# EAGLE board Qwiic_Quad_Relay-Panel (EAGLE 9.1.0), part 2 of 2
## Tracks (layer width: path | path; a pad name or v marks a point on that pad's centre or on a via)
3.3V  (via drill 0.35)
  Top 0.254: J3.2 13.6,43.04 v13.84,42.8
  Top 0.305: J2.2 83.32,42.04 v82.93,41.66
  Bottom 0.305: v13.84,42.8 13.84,39.24 16.26,36.83 17.78,36.83 18.41,37.46 33.78,37.46 34.42,36.83 36.07,36.83 37.34,38.1 53.59,38.1 55.37,36.32 56.77,36.32 58.29,37.85 74.68,37.85 75.69,36.83 79.5,36.83 82.93,40.26 v82.93,41.66
3.3V1  (via drill 0.35)
  Top 0.254: J11.2 96.66,43.04 v96.9,42.8
  Top 0.305: J10.2 166.38,42.04 v165.99,41.66
  Bottom 0.305: v96.9,42.8 96.9,39.24 99.31,36.83 100.84,36.83 101.47,37.46 116.84,37.46 117.48,36.83 119.13,36.83 120.4,38.1 136.65,38.1 138.43,36.32 139.83,36.32 141.35,37.85 157.73,37.85 158.75,36.83 162.56,36.83 165.99,40.26 v165.99,41.66
3.3V2  (via drill 0.35)
  Top 0.254: J20.2 13.6,90.54 v13.84,90.3
  Top 0.305: J19.2 83.32,89.54 v82.93,89.15
  Bottom 0.305: v13.84,90.3 13.84,86.74 16.26,84.33 17.78,84.33 18.41,84.96 33.78,84.96 34.42,84.33 36.07,84.33 37.34,85.6 53.59,85.6 55.37,83.82 56.77,83.82 58.29,85.34 74.68,85.34 75.69,84.33 79.5,84.33 82.93,87.76 v82.93,89.15
3.3V3  (via drill 0.35)
  Top 0.254: J29.2 96.66,90.54 v96.9,90.3
  Top 0.305: J28.2 166.38,89.54 v165.99,89.15
  Bottom 0.305: v96.9,90.3 96.9,86.74 99.31,84.33 100.84,84.33 101.47,84.96 116.84,84.96 117.48,84.33 119.13,84.33 120.4,85.6 136.65,85.6 138.43,83.82 139.83,83.82 141.35,85.34 157.73,85.34 158.75,84.33 162.56,84.33 165.99,87.76 v165.99,89.15
5V  (via drill 0.51)
  Top 0.254: 61.23,38.1 52.16,38.1 | 52.16,38.1 44.45,38.1 | R8.1 44.45,38.61 44.45,38.35 44.45,38.1 | 22.35,38.61 13.21,38.61 12.66,38.06 R1.2 | D9.A 83.31,37.72 82.42,38.61 72.77,38.61 72.52,38.35 72.48,38.31 72.48,37.97 | D2.A 22.35,38.61 | J4.2 35.05,43.56 34.16,42.67 U5.1 34.2,41.99 C1.1 34.2,38.65 34.16,38.61 | D3.A 64.39,50.93 64.14,50.67 64.14,47.5 64.01,47.37 | U1.2 59.56,41.95 | 59.56,41.95 R6.2 | 59.56,41.95 59.6,41.91 60.58,41.91 61.23,41.26 61.23,38.61 61.23,38.35 61.23,38.1 | R14.2 72.48,37.97 | R13.2 52.16,38.1 | 44.45,38.1 42.67,38.1 | 42.67,38.1 36.2,38.1 35.69,38.61 34.16,38.61 | 34.16,38.61 31.88,38.61 | 31.88,38.61 31.75,38.61 | 31.75,38.61 28.57,38.61 28.07,38.1 24.13,38.1 23.62,38.61 22.35,38.61 | R12.2 31.84,38.52 31.75,38.61 | 31.88,38.61 31.84,38.65 R5.2 | D7.A 42.67,38.1 | 61.23,38.1 62.99,38.1 | 62.99,38.1 63.25,38.1 64.01,37.34 70.48,37.34 70.99,37.85 72.35,37.85 72.48,37.97 | D8.A 62.99,38.1
  Top 0.508: C3.1 C2.1 66.08,47.37 64.01,47.37 60.83,47.37 v60.26,46.8 59.56,46.1 U1.2
  Bottom 0.254: J1.3 34.16,49.4 34.16,46.35 35.69,44.83 35.69,43.81 J4.2
  Bottom 0.508: JP7.2 63.75,43.31 v60.26,46.8
5V1  (via drill 0.51)
  Top 0.254: 144.28,38.1 135.22,38.1 | 135.22,38.1 127.51,38.1 | R21.1 127.51,38.61 127.51,38.35 127.51,38.1 | 105.41,38.61 96.27,38.61 95.72,38.06 R18.2 | D19.A 166.37,37.72 165.48,38.61 155.83,38.61 155.58,38.35 155.54,38.31 155.54,37.97 | D12.A 105.41,38.61 | J12.2 118.11,43.56 117.22,42.67 U7.1 117.26,41.99 C5.1 117.26,38.65 117.22,38.61 | D13.A 147.45,50.93 147.19,50.67 147.19,47.5 147.07,47.37 | U8.2 142.62,41.95 | 142.62,41.95 R33.2 | 142.62,41.95 142.66,41.91 143.64,41.91 144.28,41.26 144.28,38.61 144.28,38.35 144.28,38.1 | R29.2 155.54,37.97 | R28.2 135.22,38.1 | 127.51,38.1 125.73,38.1 | 125.73,38.1 119.25,38.1 118.75,38.61 117.22,38.61 | 117.22,38.61 114.94,38.61 | 114.94,38.61 114.81,38.61 | 114.81,38.61 111.63,38.61 111.12,38.1 107.19,38.1 106.68,38.61 105.41,38.61 | R27.2 114.9,38.52 114.81,38.61 | 114.94,38.61 114.9,38.65 R20.2 | D17.A 125.73,38.1 | 144.28,38.1 146.05,38.1 | 146.05,38.1 146.3,38.1 147.07,37.34 153.54,37.34 154.05,37.85 155.41,37.85 155.54,37.97 | D18.A 146.05,38.1
  Top 0.508: C7.1 C6.1 149.14,47.37 147.07,47.37 143.89,47.37 v143.32,46.8 142.62,46.1 U8.2
  Bottom 0.254: J14.3 117.22,49.4 117.22,46.35 118.75,44.83 118.75,43.81 J12.2
  Bottom 0.508: JP18.2 146.81,43.31 v143.32,46.8
5V2  (via drill 0.51)
  Top 0.254: 61.23,85.6 52.16,85.6 | 52.16,85.6 44.45,85.6 | R38.1 44.45,86.11 44.45,85.85 44.45,85.6 | 22.35,86.11 13.21,86.11 12.66,85.56 R35.2 | D29.A 83.31,85.22 82.42,86.11 72.77,86.11 72.52,85.85 72.48,85.81 72.48,85.47 | D22.A 22.35,86.11 | J21.2 35.05,91.06 34.16,90.17 U11.1 34.2,89.49 C9.1 34.2,86.15 34.16,86.11 | D23.A 64.39,98.42 64.14,98.17 64.14,95 64.01,94.87 | U12.2 59.56,89.45 | 59.56,89.45 R50.2 | 59.56,89.45 59.6,89.41 60.58,89.41 61.23,88.76 61.23,86.11 61.23,85.85 61.23,85.6 | R46.2 72.48,85.47 | R45.2 52.16,85.6 | 44.45,85.6 42.67,85.6 | 42.67,85.6 36.2,85.6 35.69,86.11 34.16,86.11 | 34.16,86.11 31.88,86.11 | 31.88,86.11 31.75,86.11 | 31.75,86.11 28.57,86.11 28.07,85.6 24.13,85.6 23.62,86.11 22.35,86.11 | R44.2 31.84,86.02 31.75,86.11 | 31.88,86.11 31.84,86.15 R37.2 | D27.A 42.67,85.6 | 61.23,85.6 62.99,85.6 | 62.99,85.6 63.25,85.6 64.01,84.84 70.48,84.84 70.99,85.34 72.35,85.34 72.48,85.47 | D28.A 62.99,85.6
  Top 0.508: C11.1 C10.1 66.08,94.87 64.01,94.87 60.83,94.87 v60.26,94.3 59.56,93.6 U12.2
  Bottom 0.254: J23.3 34.16,96.9 34.16,93.85 35.69,92.33 35.69,91.31 J21.2
  Bottom 0.508: JP27.2 63.75,90.81 v60.26,94.3
5V3  (via drill 0.51)
  Top 0.254: 144.28,85.6 135.22,85.6 | 135.22,85.6 127.51,85.6 | R55.1 127.51,86.11 127.51,85.85 127.51,85.6 | 105.41,86.11 96.27,86.11 95.72,85.56 R52.2 | D39.A 166.37,85.22 165.48,86.11 155.83,86.11 155.58,85.85 155.54,85.81 155.54,85.47 | D32.A 105.41,86.11 | J30.2 118.11,91.06 117.22,90.17 U15.1 117.26,89.49 C13.1 117.26,86.15 117.22,86.11 | D33.A 147.45,98.42 147.19,98.17 147.19,95 147.07,94.87 | U16.2 142.62,89.45 | 142.62,89.45 R67.2 | 142.62,89.45 142.66,89.41 143.64,89.41 144.28,88.76 144.28,86.11 144.28,85.85 144.28,85.6 | R63.2 155.54,85.47 | R62.2 135.22,85.6 | 127.51,85.6 125.73,85.6 | 125.73,85.6 119.25,85.6 118.75,86.11 117.22,86.11 | 117.22,86.11 114.94,86.11 | 114.94,86.11 114.81,86.11 | 114.81,86.11 111.63,86.11 111.12,85.6 107.19,85.6 106.68,86.11 105.41,86.11 | R61.2 114.9,86.02 114.81,86.11 | 114.94,86.11 114.9,86.15 R54.2 | D37.A 125.73,85.6 | 144.28,85.6 146.05,85.6 | 146.05,85.6 146.3,85.6 147.07,84.84 153.54,84.84 154.05,85.34 155.41,85.34 155.54,85.47 | D38.A 146.05,85.6
  Top 0.508: C15.1 C14.1 149.14,94.87 147.07,94.87 143.89,94.87 v143.32,94.3 142.62,93.6 U16.2
  Bottom 0.254: J32.3 117.22,96.9 117.22,93.85 118.75,92.33 118.75,91.31 J30.2
  Bottom 0.508: JP36.2 146.81,90.81 v143.32,94.3
!RESET
  Top 0.254: U5.4 37.97,42.41 37.08,43.3 37.08,44.2 38.35,45.47 39.88,45.47 J4.5 44.28,46.1 R8.2
!RESET1
  Top 0.254: U7.4 121.03,42.41 120.14,43.3 120.14,44.2 121.41,45.47 122.94,45.47 J12.5 127.34,46.1 R21.2
!RESET2
  Top 0.254: U11.4 37.97,89.91 37.08,90.8 37.08,91.69 38.35,92.96 39.88,92.96 J21.5 44.28,93.6 R38.2
!RESET3
  Top 0.254: U15.4 121.03,89.91 120.14,90.8 120.14,91.69 121.41,92.96 122.94,92.96 J30.5 127.34,93.6 R55.2
COM1
  Top 1.778: K1.4 13.21,20.83 15.24,18.8 15.75,18.8 20.45,18.8 23.5,15.75 J5.2
  Bottom 1.778: K1.4 13.21,20.83 15.24,18.8 20.49,18.8 J5.2
COM2
  Top 1.778: K2.4 33.53,20.32 35.31,18.54 37.13,18.54 J6.2
  Bottom 1.778: K2.4 33.53,20.32 35.31,18.54 37.13,18.54 J6.2 | J6.2
COM3
  Top 1.778: K3.4 53.85,18.29 56.31,15.83 J7.2
  Bottom 1.778: K3.4 53.85,18.29 56.31,15.83 J7.2
COM4
  Top 1.778: K4.4 74.17,17.23 J8.2 | K4.4
  Bottom 1.778: K4.4 74.17,17.23 J8.2 | K4.4
COM5
  Top 1.778: K5.4 96.27,20.83 98.3,18.8 98.81,18.8 103.51,18.8 106.55,15.75 J13.2
  Bottom 1.778: K5.4 96.27,20.83 98.3,18.8 103.55,18.8 J13.2
COM6
  Top 1.778: K6.4 116.59,20.32 118.36,18.54 120.19,18.54 J15.2
  Bottom 1.778: K6.4 116.59,20.32 118.36,18.54 120.19,18.54 J15.2 | J15.2
COM7
  Top 1.778: K7.4 136.91,18.29 139.37,15.83 J16.2
  Bottom 1.778: K7.4 136.91,18.29 139.37,15.83 J16.2
COM8
  Top 1.778: K8.4 157.23,17.23 J17.2 | K8.4
  Bottom 1.778: K8.4 157.23,17.23 J17.2 | K8.4
COM9
  Top 1.778: K9.4 13.21,68.33 15.24,66.29 15.75,66.29 20.45,66.29 23.5,63.25 J22.2
  Bottom 1.778: K9.4 13.21,68.33 15.24,66.29 20.49,66.29 J22.2
COM10
  Top 1.778: K10.4 33.53,67.82 35.31,66.04 37.13,66.04 J24.2
  Bottom 1.778: K10.4 33.53,67.82 35.31,66.04 37.13,66.04 J24.2 | J24.2
COM11
  Top 1.778: K11.4 53.85,65.79 56.31,63.33 J25.2
  Bottom 1.778: K11.4 53.85,65.79 56.31,63.33 J25.2
COM12
  Top 1.778: K12.4 74.17,64.72 J26.2 | K12.4
  Bottom 1.778: K12.4 74.17,64.72 J26.2 | K12.4
COM13
  Top 1.778: K13.4 96.27,68.33 98.3,66.29 98.81,66.29 103.51,66.29 106.55,63.25 J31.2
  Bottom 1.778: K13.4 96.27,68.33 98.3,66.29 103.55,66.29 J31.2
COM14
  Top 1.778: K14.4 116.59,67.82 118.36,66.04 120.19,66.04 J33.2
  Bottom 1.778: K14.4 116.59,67.82 118.36,66.04 120.19,66.04 J33.2 | J33.2
COM15
  Top 1.778: K15.4 136.91,65.79 139.37,63.33 J34.2
  Bottom 1.778: K15.4 136.91,65.79 139.37,63.33 J34.2
COM16
  Top 1.778: K16.4 157.23,64.72 J35.2 | K16.4
  Bottom 1.778: K16.4 157.23,64.72 J35.2 | K16.4
GND  (via drill 0.3)
  other vias: 53.34,36.96 73.53,36.83 32.77,36.45 13.97,37.34 71.37,36.83 86.11,37.08 50.8,36.96 11.43,37.34 30.86,36.45 38.48,40.64
  pour Bottom: 6.86,32.77 89.41,32.77 89.41,53.85 6.86,53.85
  pour Top: 6.86,32.77 6.86,53.85 89.41,53.85 89.41,32.77
GND1  (via drill 0.3)
  other vias: 136.4,36.96 156.59,36.83 115.82,36.45 97.03,37.34 154.43,36.83 169.16,37.08 133.86,36.96 94.49,37.34 113.92,36.45 121.54,40.64
  pour Bottom: 89.92,32.77 172.47,32.77 172.47,53.85 89.92,53.85
  pour Top: 89.92,32.77 89.92,53.85 172.47,53.85 172.47,32.77
GND2  (via drill 0.3)
  other vias: 53.34,84.45 73.53,84.33 32.77,83.95 13.97,84.84 71.37,84.33 86.11,84.58 50.8,84.45 11.43,84.84 30.86,83.95 38.48,88.14
  pour Bottom: 6.86,80.26 89.41,80.26 89.41,101.35 6.86,101.35
  pour Top: 6.86,80.26 6.86,101.35 89.41,101.35 89.41,80.26
GND3  (via drill 0.3)
  other vias: 136.4,84.45 156.59,84.33 115.82,83.95 97.03,84.84 154.43,84.33 169.16,84.58 133.86,84.45 94.49,84.84 113.92,83.95 121.54,88.14
  pour Bottom: 89.92,80.26 172.47,80.26 172.47,101.35 89.92,101.35
  pour Top: 89.92,80.26 89.92,101.35 172.47,101.35 172.47,80.26
MISO  (via drill 0.35)
  Top 0.254: U5.8 v41.78,49.02
  Bottom 0.254: v41.78,49.02 40,47.24 35.94,47.24 35.43,46.74 J4.1
MISO1  (via drill 0.35)
  Top 0.254: U7.8 v124.84,49.02
  Bottom 0.254: v124.84,49.02 123.06,47.24 119,47.24 118.49,46.74 J12.1
MISO2  (via drill 0.35)
  Top 0.254: U11.8 v41.78,96.52
  Bottom 0.254: v41.78,96.52 40,94.74 35.94,94.74 35.43,94.23 J21.1
MISO3  (via drill 0.35)
  Top 0.254: U15.8 v124.84,96.52
  Bottom 0.254: v124.84,96.52 123.06,94.74 119,94.74 118.49,94.23 J30.1
N$1
  Top 0.254: K2.5 41.4,22.1 38.61,24.89 38.61,31.88 37.85,32.64 37.72,32.77 30.1,32.77 29.84,33.03 D6.C 29.84,34.75 R12.1
N$2
  Top 0.254: D1.A 15.58,33.53 Q4.3 15.92,33.53 R4.1 25.06,30.57 K1.1
N$3
  Top 0.254: U3.3 25.27,44.45 25.65,44.07 27.94,44.07 28.96,43.05 31.5,43.05 31.88,43.43 R11.1
N$4
  Top 0.508: U1.3 61.87,41.25 62.99,40.13 63.63,39.5 D11.C 65.16,40.78 65.53,41.15 C4.A
N$5
  Top 0.254: R10.1 28.66,44.11 27.81,44.96 U3.1
N$6  (via drill 0.35)
  Top 0.254: U3.6 25.27,43.31 25.53,43.56 27.56,43.56 27.81,43.31 U3.8 27.81,41.27 28.57,40.51 v28.96,40.51 R5.1 | 51.94,43.18 53.85,43.18 54.1,43.18 54.48,42.8 U2.8 | U2.6 51.94,43.18 | v48.39,40.64 48.39,41.4 50.16,43.18 51.94,43.18
  Bottom 0.254: v48.39,40.64 47.75,40 29.46,40 v28.96,40.51
N$7
  Top 0.254: R1.1 10.79,34.88 D1.C 10.79,33.03 11.05,32.77 17.65,32.77 18.29,32.13 18.29,25.4 19.05,24.64 23.37,24.64 K1.5
N$8
  Top 0.254: R4.2 26.79,33.55 26.79,34.17 26.54,34.42 22.61,34.42 22.35,34.67 D2.C
N$9
  Top 0.254: U2.1 54.48,44.45 53.72,43.69 49.91,43.69 49.02,42.8 47.12,42.8 46.48,43.43 R2.1
N$10
  Top 0.254: D10.A 98.64,33.53 Q5.3 98.98,33.53 R19.1 108.12,30.57 K5.1
N$11
  Top 0.254: U2.3 51.94,45.08 51.09,44.23 R3.1
N$12
  Top 0.254: K2.1 45.38,30.57 R15.1 34.97,33.53 Q3.3 34.63,33.53 D6.A
N$13
  Top 0.254: D3.C 67.82,50.91 67.82,50.04 67.69,49.91 66.42,49.91 66.21,49.7 R9.1
N$14
  Top 0.254: R13.1 50.16,34.75 D4.C 50.16,33.03 50.42,32.77 58.04,32.77 58.93,31.88 | 58.93,31.88 58.93,23.5 60.26,22.16 60.32,22.1 K3.5 | 58.93,31.88 arc90 58.93,31.88
N$15
  Top 0.254: D4.A 54.95,33.53 Q2.3 55.29,33.53 R16.1 65.7,30.57 K3.1
N$16
  Top 0.254: 79.12,23.5 80.52,22.1 K4.5 | R14.1 70.48,34.88 D5.C 70.48,33.02 70.74,32.77 78.49,32.77 79.12,32.13 79.12,23.5 | 79.12,23.5
N$17
  Top 0.254: D5.A 75.27,33.53 Q1.3 75.61,33.53 R17.1 86.02,29.72 K4.1
N$18
  Top 0.254: R18.1 93.85,34.88 D10.C 93.85,33.03 94.11,32.77 100.71,32.77 101.35,32.13 101.35,25.4 102.11,24.64 106.43,24.64 K5.5
N$19
  Top 0.254: U1.1 57.25,43.24 57.82,42.67 R6.1 R7.2
N$20
  Top 0.254: R17.2 87.75,33.55 87.76,33.57 87.76,34.16 87.5,34.42 83.57,34.42 83.31,34.67 D9.C
N$21
  Top 0.254: R16.2 67.42,33.55 67.42,34.17 67.18,34.42 63.25,34.42 62.99,34.67 D8.C
N$22
  Top 0.254: D7.C 42.67,34.67 42.93,34.42 46.86,34.42 47.08,34.2 R15.2
N$23
  Top 0.254: R19.2 109.84,33.55 109.84,34.17 109.6,34.42 105.66,34.42 105.41,34.67 D12.C
N$24
  Top 0.254: D13.C 150.88,50.91 150.88,50.04 150.75,49.91 149.48,49.91 149.26,49.7 R22.1
N$25
  Top 0.254: U4.3 108.33,44.45 108.71,44.07 111,44.07 112.01,43.05 114.55,43.05 114.94,43.43 R26.1
N$26
  Top 0.254: R25.1 111.72,44.11 110.87,44.96 U4.1
N$27  (via drill 0.35)
  Top 0.254: U4.6 108.33,43.31 108.59,43.56 110.62,43.56 110.87,43.31 U4.8 110.87,41.27 111.63,40.51 v112.01,40.51 R20.1 | 135,43.18 136.91,43.18 137.16,43.18 137.54,42.8 U6.8 | U6.6 135,43.18 | v131.44,40.64 131.44,41.4 133.22,43.18 135,43.18
  Bottom 0.254: v131.44,40.64 130.81,40 112.52,40 v112.01,40.51
N$28
  Top 0.254: U6.1 137.54,44.45 136.78,43.69 132.97,43.69 132.08,42.8 130.17,42.8 129.54,43.43 R23.1
N$29
  Top 0.254: U6.3 135,45.08 134.15,44.23 R24.1
N$30
  Top 0.254: K6.5 124.46,22.1 121.67,24.89 121.67,31.88 120.9,32.64 120.78,32.77 113.16,32.77 112.9,33.03 D16.C 112.9,34.75 R27.1
N$31
  Top 0.254: K6.1 128.44,30.57 R30.1 118.03,33.53 Q8.3 117.69,33.53 D16.A
N$32
  Top 0.254: R28.1 133.22,34.75 D14.C 133.22,33.03 133.48,32.77 141.1,32.77 141.99,31.88 | 141.99,31.88 141.99,23.5 143.32,22.16 143.38,22.1 K7.5 | 141.99,31.88 arc90 141.99,31.88
N$33
  Top 0.254: D14.A 138.01,33.53 Q7.3 138.35,33.53 R31.1 148.76,30.57 K7.1
N$34
  Top 0.254: 162.18,23.5 163.58,22.1 K8.5 | R29.1 153.54,34.88 D15.C 153.54,33.02 153.8,32.77 161.54,32.77 162.18,32.13 162.18,23.5 | 162.18,23.5
N$35
  Top 0.254: D15.A 158.33,33.53 Q6.3 158.67,33.53 R32.1 169.08,29.72 K8.1
N$36
  Top 0.254: R32.2 170.8,33.55 170.81,33.57 170.81,34.16 170.56,34.42 166.62,34.42 166.37,34.67 D19.C
N$37
  Top 0.254: R31.2 150.48,33.55 150.48,34.17 150.24,34.42 146.3,34.42 146.05,34.67 D18.C
N$38
  Top 0.254: D17.C 125.73,34.67 125.98,34.42 129.92,34.42 130.14,34.2 R30.2
N$39
  Top 0.254: U8.1 140.31,43.24 140.88,42.67 R33.1 R34.2
N$40
  Top 0.508: U8.3 144.93,41.25 146.05,40.13 146.69,39.5 D20.C 148.22,40.78 148.59,41.15 C8.A
N$41
  Top 0.254: D21.A 15.58,81.03 Q9.3 15.92,81.03 R36.1 25.06,78.07 K9.1
N$42
  Top 0.254: R35.1 10.79,82.38 D21.C 10.79,80.53 11.05,80.26 17.65,80.26 18.29,79.63 18.29,72.9 19.05,72.14 23.37,72.14 K9.5
N$43
  Top 0.254: R36.2 26.79,81.05 26.79,81.67 26.54,81.92 22.61,81.92 22.35,82.17 D22.C
N$44
  Top 0.254: D23.C 67.82,98.41 67.82,97.54 67.69,97.41 66.42,97.41 66.21,97.19 R39.1
N$45
  Top 0.254: U9.3 25.27,91.95 25.65,91.57 27.94,91.57 28.96,90.55 31.5,90.55 31.88,90.93 R43.1
N$46
  Top 0.254: R42.1 28.66,91.61 27.81,92.46 U9.1
N$47  (via drill 0.35)
  Top 0.254: U9.6 25.27,90.81 25.53,91.06 27.56,91.06 27.81,90.81 U9.8 27.81,88.77 28.57,88.01 v28.96,88.01 R37.1 | 51.94,90.68 53.85,90.68 54.1,90.68 54.48,90.3 U10.8 | U10.6 51.94,90.68 | v48.39,88.14 48.39,88.9 50.16,90.68 51.94,90.68
  Bottom 0.254: v48.39,88.14 47.75,87.5 29.46,87.5 v28.96,88.01
N$48
  Top 0.254: U10.1 54.48,91.95 53.72,91.19 49.91,91.19 49.02,90.3 47.12,90.3 46.48,90.93 R40.1
N$49
  Top 0.254: U10.3 51.94,92.58 51.09,91.73 R41.1
N$50
  Top 0.254: K10.5 41.4,69.6 38.61,72.39 38.61,79.38 37.85,80.14 37.72,80.26 30.1,80.26 29.84,80.53 D26.C 29.84,82.25 R44.1
N$51
  Top 0.254: K10.1 45.38,78.07 R47.1 34.97,81.03 Q12.3 34.63,81.03 D26.A
N$52
  Top 0.254: R45.1 50.16,82.25 D24.C 50.16,80.53 50.42,80.26 58.04,80.26 58.93,79.38 | 58.93,79.38 58.93,70.99 60.26,69.66 60.32,69.6 K11.5 | 58.93,79.38 arc90 58.93,79.38
N$53
  Top 0.254: D24.A 54.95,81.03 Q11.3 55.29,81.03 R48.1 65.7,78.07 K11.1
N$54
  Top 0.254: 79.12,70.99 80.52,69.6 K12.5 | R46.1 70.48,82.38 D25.C 70.48,80.52 70.74,80.26 78.49,80.26 79.12,79.63 79.12,70.99 | 79.12,70.99
N$55
  Top 0.254: D25.A 75.27,81.03 Q10.3 75.61,81.03 R49.1 86.02,77.22 K12.1
N$56
  Top 0.254: R49.2 87.75,81.05 87.76,81.06 87.76,81.66 87.5,81.92 83.57,81.92 83.31,82.17 D29.C
N$57
  Top 0.254: R48.2 67.42,81.05 67.42,81.67 67.18,81.92 63.25,81.92 62.99,82.17 D28.C
N$58
  Top 0.254: D27.C 42.67,82.17 42.93,81.92 46.86,81.92 47.08,81.7 R47.2
N$59
  Top 0.254: U12.1 57.25,90.74 57.82,90.17 R50.1 R51.2
N$60
  Top 0.508: U12.3 61.87,88.75 62.99,87.63 63.63,87 D30.C 65.16,88.27 65.53,88.65 C12.A
N$61
  Top 0.254: D31.A 98.64,81.03 Q13.3 98.98,81.03 R53.1 108.12,78.07 K13.1
N$62
  Top 0.254: R52.1 93.85,82.38 D31.C 93.85,80.53 94.11,80.26 100.71,80.26 101.35,79.63 101.35,72.9 102.11,72.14 106.43,72.14 K13.5
N$63
  Top 0.254: R53.2 109.84,81.05 109.84,81.67 109.6,81.92 105.66,81.92 105.41,82.17 D32.C
N$64
  Top 0.254: D33.C 150.88,98.41 150.88,97.54 150.75,97.41 149.48,97.41 149.26,97.19 R56.1
N$65
  Top 0.254: U13.3 108.33,91.95 108.71,91.57 111,91.57 112.01,90.55 114.55,90.55 114.94,90.93 R60.1
N$66
  Top 0.254: R59.1 111.72,91.61 110.87,92.46 U13.1
N$67  (via drill 0.35)
  Top 0.254: U13.6 108.33,90.81 108.59,91.06 110.62,91.06 110.87,90.81 U13.8 110.87,88.77 111.63,88.01 v112.01,88.01 R54.1 | 135,90.68 136.91,90.68 137.16,90.68 137.54,90.3 U14.8 | U14.6 135,90.68 | v131.44,88.14 131.44,88.9 133.22,90.68 135,90.68
  Bottom 0.254: v131.44,88.14 130.81,87.5 112.52,87.5 v112.01,88.01
N$68
  Top 0.254: U14.1 137.54,91.95 136.78,91.19 132.97,91.19 132.08,90.3 130.17,90.3 129.54,90.93 R57.1
N$69
  Top 0.254: U14.3 135,92.58 134.15,91.73 R58.1
N$70
  Top 0.254: K14.5 124.46,69.6 121.67,72.39 121.67,79.38 120.9,80.14 120.78,80.26 113.16,80.26 112.9,80.53 D36.C 112.9,82.25 R61.1
N$71
  Top 0.254: K14.1 128.44,78.07 R64.1 118.03,81.03 Q16.3 117.69,81.03 D36.A
N$72
  Top 0.254: R62.1 133.22,82.25 D34.C 133.22,80.53 133.48,80.26 141.1,80.26 141.99,79.38 | 141.99,79.38 141.99,70.99 143.32,69.66 143.38,69.6 K15.5 | 141.99,79.38 arc90 141.99,79.38
N$73
  Top 0.254: D34.A 138.01,81.03 Q15.3 138.35,81.03 R65.1 148.76,78.07 K15.1
N$74
  Top 0.254: 162.18,70.99 163.58,69.6 K16.5 | R63.1 153.54,82.38 D35.C 153.54,80.52 153.8,80.26 161.54,80.26 162.18,79.63 162.18,70.99 | 162.18,70.99
N$75
  Top 0.254: D35.A 158.33,81.03 Q14.3 158.67,81.03 R66.1 169.08,77.22 K16.1
N$76
  Top 0.254: R66.2 170.8,81.05 170.81,81.06 170.81,81.66 170.56,81.92 166.62,81.92 166.37,82.17 D39.C
N$77
  Top 0.254: R65.2 150.48,81.05 150.48,81.67 150.24,81.92 146.3,81.92 146.05,82.17 D38.C
N$78
  Top 0.254: D37.C 125.73,82.17 125.98,81.92 129.92,81.92 130.14,81.7 R64.2
N$79
  Top 0.254: U16.1 140.31,90.74 140.88,90.17 R67.1 R68.2
N$80
  Top 0.508: U16.3 144.93,88.75 146.05,87.63 146.69,87 D40.C 148.22,88.27 148.59,88.65 C16.A
NC1
  Top 1.778: K1.2 22.19,22.1 J5.3
  Bottom 1.778: K1.2 22.17,22.1 28.52,15.75 J5.3
NC2
  Top 1.778: K2.2 38.61,22.1 44.92,15.78 J6.3
  Bottom 1.778: K2.2 38.57,22.1 J6.3
NC3
  Top 1.778: K3.2 61.34,17.14 61.34,15.78 J7.3
  Bottom 1.778: K3.2 61.31,17.18 J7.3
NC4
  Top 1.778: K4.2 77.72,21.08 77.72,15.78 J8.3
  Bottom 1.778: K4.2 77.69,21.11 J8.3
NC5
  Top 1.778: K5.2 105.25,22.1 J13.3
  Bottom 1.778: K5.2 105.23,22.1 111.58,15.75 J13.3
NC6
  Top 1.778: K6.2 121.67,22.1 127.98,15.78 J15.3
  Bottom 1.778: K6.2 121.63,22.1 J15.3
NC7
  Top 1.778: K7.2 144.4,17.14 144.4,15.78 J16.3
  Bottom 1.778: K7.2 144.37,17.18 J16.3
NC8
  Top 1.778: K8.2 160.78,21.08 160.78,15.78 J17.3
  Bottom 1.778: K8.2 160.75,21.11 J17.3
NC9
  Top 1.778: K9.2 22.19,69.6 J22.3
  Bottom 1.778: K9.2 22.17,69.6 28.52,63.25 J22.3
NC10
  Top 1.778: K10.2 38.61,69.6 44.92,63.28 J24.3
  Bottom 1.778: K10.2 38.57,69.6 J24.3
NC11
  Top 1.778: K11.2 61.34,64.64 61.34,63.28 J25.3
  Bottom 1.778: K11.2 61.31,64.68 J25.3
NC12
  Top 1.778: K12.2 77.72,68.58 77.72,63.28 J26.3
  Bottom 1.778: K12.2 77.69,68.61 J26.3
NC13
  Top 1.778: K13.2 105.25,69.6 J31.3
  Bottom 1.778: K13.2 105.23,69.6 111.58,63.25 J31.3
NC14
  Top 1.778: K14.2 121.67,69.6 127.98,63.28 J33.3
  Bottom 1.778: K14.2 121.63,69.6 J33.3
NC15
  Top 1.778: K15.2 144.4,64.64 144.4,63.28 J34.3
  Bottom 1.778: K15.2 144.37,64.68 J34.3
NC16
  Top 1.778: K16.2 160.78,68.58 160.78,63.28 J35.3
  Bottom 1.778: K16.2 160.75,68.61 J35.3
NO1
  Top 1.778: K1.3 10.67,18.29 13.21,15.75 J5.1
  Bottom 1.778: J5.1 13.21,15.75 10.67,18.29 K1.3
NO2
  Top 1.778: J6.1 33.66,15.75 30.99,18.41 K2.3
  Bottom 1.778: J6.1 33.66,15.75 30.99,18.41 K2.3
NO3
  Top 1.778: J7.1 K3.3
  Bottom 1.778: J7.1 K3.3
NO4
  Top 1.778: J8.1 67.69,18.16 K4.3
  Bottom 1.778: J8.1 67.69,18.16 K4.3
NO5
  Top 1.778: K5.3 93.73,18.29 96.27,15.75 J13.1
  Bottom 1.778: J13.1 96.27,15.75 93.73,18.29 K5.3
NO6
  Top 1.778: J15.1 116.71,15.75 114.05,18.41 K6.3
  Bottom 1.778: J15.1 116.71,15.75 114.05,18.41 K6.3
NO7
  Top 1.778: J16.1 K7.3
  Bottom 1.778: J16.1 K7.3
NO8
  Top 1.778: J17.1 150.75,18.16 K8.3
  Bottom 1.778: J17.1 150.75,18.16 K8.3
NO9
  Top 1.778: K9.3 10.67,65.79 13.21,63.25 J22.1
  Bottom 1.778: J22.1 13.21,63.25 10.67,65.79 K9.3
NO10
  Top 1.778: J24.1 33.66,63.25 30.99,65.91 K10.3
  Bottom 1.778: J24.1 33.66,63.25 30.99,65.91 K10.3
NO11
  Top 1.778: J25.1 K11.3
  Bottom 1.778: J25.1 K11.3
NO12
  Top 1.778: J26.1 67.69,65.66 K12.3
  Bottom 1.778: J26.1 67.69,65.66 K12.3
NO13
  Top 1.778: K13.3 93.73,65.79 96.27,63.25 J31.1
  Bottom 1.778: J31.1 96.27,63.25 93.73,65.79 K13.3
NO14
  Top 1.778: J33.1 116.71,63.25 114.05,65.91 K14.3
  Bottom 1.778: J33.1 116.71,63.25 114.05,65.91 K14.3
NO15
  Top 1.778: J34.1 K15.3
  Bottom 1.778: J34.1 K15.3
NO16
  Top 1.778: J35.1 150.75,65.66 K16.3
  Bottom 1.778: J35.1 150.75,65.66 K16.3
OPTO_1  (via drill 0.35)
  Top 0.254: Q4.1 16.7,37.02 v17.4,37.72 | U3.5 24,41.02 v24.13,40.89
  Bottom 0.254: v17.4,37.72 17.78,38.1 25.4,38.1 25.91,38.61 25.91,39.88 24.89,40.89 v24.13,40.89
OPTO_2  (via drill 0.35)
  Top 0.254: v26.54,40.89 U3.7 | v35.05,37.72 35.43,37.72 35.75,37.4 Q3.1
  Bottom 0.254: v26.54,40.89 26.54,38.48 26.92,38.1 34.67,38.1 v35.05,37.72
OPTO_3  (via drill 0.35)
  Top 0.254: U2.5 50.67,41.53 51.18,41.02 52.7,41.02 v52.96,40.77 | Q2.1 56.07,37.02 v55.88,37.21
  Bottom 0.305: v52.96,40.77 53.97,39.75 53.97,38.73 55.5,37.21 v55.88,37.21
OPTO_4  (via drill 0.35)
  Top 0.254: Q1.1 76.39,37.53 v76.2,37.72 | U2.7 53.34,42.16 53.34,41.78 v54.36,40.77
  Bottom 0.254: v76.2,37.72 75.44,38.48 55.24,38.48 54.61,39.12 54.61,40.51 v54.36,40.77
OPTO_5  (via drill 0.35)
  Top 0.254: Q5.1 99.76,37.02 v100.46,37.72 | U4.5 107.06,41.02 v107.19,40.89
  Bottom 0.254: v100.46,37.72 100.84,38.1 108.46,38.1 108.97,38.61 108.97,39.88 107.95,40.89 v107.19,40.89
OPTO_6  (via drill 0.35)
  Top 0.254: v109.6,40.89 U4.7 | v118.11,37.72 118.49,37.72 118.81,37.4 Q8.1
  Bottom 0.254: v109.6,40.89 109.6,38.48 109.98,38.1 117.73,38.1 v118.11,37.72
OPTO_7  (via drill 0.35)
  Top 0.254: U6.5 133.73,41.53 134.24,41.02 135.76,41.02 v136.02,40.77 | Q7.1 139.13,37.02 v138.94,37.21
  Bottom 0.305: v136.02,40.77 137.03,39.75 137.03,38.73 138.56,37.21 v138.94,37.21
OPTO_8  (via drill 0.35)
  Top 0.254: Q6.1 159.45,37.53 v159.26,37.72 | U6.7 136.4,42.16 136.4,41.78 v137.41,40.77
  Bottom 0.254: v159.26,37.72 158.5,38.48 138.3,38.48 137.67,39.12 137.67,40.51 v137.41,40.77
OPTO_9  (via drill 0.35)
  Top 0.254: Q9.1 16.7,84.52 v17.4,85.22 | U9.5 24,88.52 v24.13,88.39
  Bottom 0.254: v17.4,85.22 17.78,85.6 25.4,85.6 25.91,86.11 25.91,87.38 24.89,88.39 v24.13,88.39
OPTO_10  (via drill 0.35)
  Top 0.254: v26.54,88.39 U9.7 | v35.05,85.22 35.43,85.22 35.75,84.9 Q12.1
  Bottom 0.254: v26.54,88.39 26.54,85.98 26.92,85.6 34.67,85.6 v35.05,85.22
OPTO_11  (via drill 0.35)
  Top 0.254: U10.5 50.67,89.03 51.18,88.52 52.7,88.52 v52.96,88.27 | Q11.1 56.07,84.52 v55.88,84.71
  Bottom 0.305: v52.96,88.27 53.97,87.25 53.97,86.23 55.5,84.71 v55.88,84.71
OPTO_12  (via drill 0.35)
  Top 0.254: Q10.1 76.39,85.03 v76.2,85.22 | U10.7 53.34,89.66 53.34,89.28 v54.36,88.27
  Bottom 0.254: v76.2,85.22 75.44,85.98 55.24,85.98 54.61,86.61 54.61,88.01 v54.36,88.27
OPTO_13  (via drill 0.35)
  Top 0.254: Q13.1 99.76,84.52 v100.46,85.22 | U13.5 107.06,88.52 v107.19,88.39
  Bottom 0.254: v100.46,85.22 100.84,85.6 108.46,85.6 108.97,86.11 108.97,87.38 107.95,88.39 v107.19,88.39
OPTO_14  (via drill 0.35)
  Top 0.254: v109.6,88.39 U13.7 | v118.11,85.22 118.49,85.22 118.81,84.9 Q16.1
  Bottom 0.254: v109.6,88.39 109.6,85.98 109.98,85.6 117.73,85.6 v118.11,85.22
OPTO_15  (via drill 0.35)
  Top 0.254: U14.5 133.73,89.03 134.24,88.52 135.76,88.52 v136.02,88.27 | Q15.1 139.13,84.52 v138.94,84.71
  Bottom 0.305: v136.02,88.27 137.03,87.25 137.03,86.23 138.56,84.71 v138.94,84.71
OPTO_16  (via drill 0.35)
  Top 0.254: Q14.1 159.45,85.03 v159.26,85.22 | U14.7 136.4,89.66 136.4,89.28 v137.41,88.27
  Bottom 0.254: v159.26,85.22 158.5,85.98 138.3,85.98 137.67,86.61 137.67,88.01 v137.41,88.27
RELAY_CTRL1
  Top 0.254: U5.10 39.24,49.15 40.26,50.16 42.42,50.16 42.93,49.66 45.08,49.66 46.48,48.26 R2.2
RELAY_CTRL2
  Top 0.254: U5.11 | U5.11 37.97,48.77 39.37,50.16 39.88,50.67 42.67,50.67 43.18,50.16 45.72,50.16 48.51,47.37 R3.2
RELAY_CTRL3
  Top 0.254: R10.2 29.97,47.62 32.13,49.78 35.81,49.78 36.7,48.89 U5.12
RELAY_CTRL4
  Top 0.254: U5.13 35.43,48.64 34.8,49.28 32.77,49.28 31.88,48.39 R11.2
RELAY_CTRL5
  Top 0.254: U7.10 122.3,49.15 123.32,50.16 125.48,50.16 125.98,49.66 128.14,49.66 129.54,48.26 R23.2
RELAY_CTRL6
  Top 0.254: U7.11 | U7.11 121.03,48.77 122.43,50.16 122.94,50.67 125.73,50.67 126.24,50.16 128.78,50.16 131.57,47.37 R24.2
RELAY_CTRL7
  Top 0.254: R25.2 113.03,47.62 115.19,49.78 118.87,49.78 119.76,48.89 U7.12
RELAY_CTRL8
  Top 0.254: U7.13 118.49,48.64 117.86,49.28 115.82,49.28 114.94,48.39 R26.2
RELAY_CTRL9
  Top 0.254: U11.10 39.24,96.65 40.26,97.66 42.42,97.66 42.93,97.16 45.08,97.16 46.48,95.76 R40.2
RELAY_CTRL10
  Top 0.254: U11.11 | U11.11 37.97,96.27 39.37,97.66 39.88,98.17 42.67,98.17 43.18,97.66 45.72,97.66 48.51,94.87 R41.2
RELAY_CTRL11
  Top 0.254: R42.2 29.97,95.12 32.13,97.28 35.81,97.28 36.7,96.39 U11.12
RELAY_CTRL12
  Top 0.254: U11.13 35.43,96.14 34.8,96.77 32.77,96.77 31.88,95.89 R43.2
RELAY_CTRL13
  Top 0.254: U15.10 122.3,96.65 123.32,97.66 125.48,97.66 125.98,97.16 128.14,97.16 129.54,95.76 R57.2
RELAY_CTRL14
  Top 0.254: U15.11 | U15.11 121.03,96.27 122.43,97.66 122.94,98.17 125.73,98.17 126.24,97.66 128.78,97.66 131.57,94.87 R58.2
RELAY_CTRL15
  Top 0.254: R59.2 113.03,95.12 115.19,97.28 118.87,97.28 119.76,96.39 U15.12
RELAY_CTRL16
  Top 0.254: U15.13 118.49,96.14 117.86,96.77 115.82,96.77 114.94,95.89 R60.2
SCL/SCK  (via drill 0.35)
  Top 0.254: J2.4 82.02,44.04 v81.66,43.69 | J4.3 39.12,46.1 40.51,47.5 U5.9 v40.51,49.02 | 55.24,40 55.12,40 | 55.12,40 51.05,40 v50.8,40 | v27.43,40 v23.37,40 | J3.4 14.07,41.04 15.11,40 v16.26,40 | 55.12,40 55.24,40 | 55.24,40 v55.63,40.39
  Bottom 0.254: v23.37,40 v16.26,40 | J1.1 42.42,51.43 40.51,49.53 v40.51,49.02 | J4.3 37.72,46.1 37.08,45.47 37.08,42.42 37.72,41.78 49.4,41.78 50.8,40.39 v50.8,40 50.8,39.75 50.55,39.5 28.19,39.5 27.69,40 v27.43,40 | v81.66,43.69 81.15,43.18 81.15,41.02 80.52,40.39 v55.63,40.39 | v27.43,40
SCL/SCK1  (via drill 0.35)
  Top 0.254: J10.4 165.08,44.04 v164.72,43.69 | J12.3 122.17,46.1 123.57,47.5 U7.9 v123.57,49.02 | 138.3,40 138.18,40 | 138.18,40 134.11,40 v133.86,40 | v110.49,40 v106.43,40 | J11.4 97.13,41.04 98.17,40 v99.31,40 | 138.18,40 138.3,40 | 138.3,40 v138.68,40.39
  Bottom 0.254: v106.43,40 v99.31,40 | J14.1 125.48,51.43 123.57,49.53 v123.57,49.02 | J12.3 120.78,46.1 120.14,45.47 120.14,42.42 120.78,41.78 132.46,41.78 133.86,40.39 v133.86,40 133.86,39.75 133.6,39.5 111.25,39.5 110.74,40 v110.49,40 | v164.72,43.69 164.21,43.18 164.21,41.02 163.58,40.39 v138.68,40.39 | v110.49,40
SCL/SCK2  (via drill 0.35)
  Top 0.254: J19.4 82.02,91.54 v81.66,91.19 | J21.3 39.12,93.6 40.51,95 U11.9 v40.51,96.52 | 55.24,87.5 55.12,87.5 | 55.12,87.5 51.05,87.5 v50.8,87.5 | v27.43,87.5 v23.37,87.5 | J20.4 14.07,88.54 15.11,87.5 v16.26,87.5 | 55.12,87.5 55.24,87.5 | 55.24,87.5 v55.63,87.88
  Bottom 0.254: v23.37,87.5 v16.26,87.5 | J23.1 42.42,98.93 40.51,97.03 v40.51,96.52 | J21.3 37.72,93.6 37.08,92.96 37.08,89.92 37.72,89.28 49.4,89.28 50.8,87.88 v50.8,87.5 50.8,87.25 50.55,87 28.19,87 27.69,87.5 v27.43,87.5 | v81.66,91.19 81.15,90.68 81.15,88.52 80.52,87.88 v55.63,87.88 | v27.43,87.5
SCL/SCK3  (via drill 0.35)
  Top 0.254: J28.4 165.08,91.54 v164.72,91.19 | J30.3 122.17,93.6 123.57,95 U15.9 v123.57,96.52 | 138.3,87.5 138.18,87.5 | 138.18,87.5 134.11,87.5 v133.86,87.5 | v110.49,87.5 v106.43,87.5 | J29.4 97.13,88.54 98.17,87.5 v99.31,87.5 | 138.18,87.5 138.3,87.5 | 138.3,87.5 v138.68,87.88
  Bottom 0.254: v106.43,87.5 v99.31,87.5 | J32.1 125.48,98.93 123.57,97.03 v123.57,96.52 | J30.3 120.78,93.6 120.14,92.96 120.14,89.92 120.78,89.28 132.46,89.28 133.86,87.88 v133.86,87.5 133.86,87.25 133.6,87 111.25,87 110.74,87.5 v110.49,87.5 | v164.72,91.19 164.21,90.68 164.21,88.52 163.58,87.88 v138.68,87.88 | v110.49,87.5
SDA/MOSI  (via drill 0.35)
  Top 0.254: v27.43,38.99 v25.02,38.99 | J1.2 39.88,51.43 40.13,51.18 43.56,51.18 v43.69,51.05 | J4.4 39.37,44.96 41.78,44.96 | 41.78,44.96 v42.8,44.96 | U5.7 41.78,44.96 | J3.3 14.34,42.04 v14.61,41.78 | v82.04,42.54 82.54,43.04 J2.3 | v56.13,39.37 55.75,38.99 v52.96,38.99
  Bottom 0.254: v25.02,38.99 15.11,38.99 14.61,39.5 v14.61,41.78 | v42.8,44.96 42.8,43.05 43.56,42.29 50.16,42.29 52.96,39.5 v52.96,38.99 49.91,38.99 v27.43,38.99 | v42.8,44.96 | v42.8,44.96 42.8,49.66 43.69,50.55 v43.69,51.05 | v82.04,42.54 82.04,40.26 81.15,39.37 v56.13,39.37
SDA/MOSI1  (via drill 0.35)
  Top 0.254: v110.49,38.99 v108.08,38.99 | J14.2 122.94,51.43 123.19,51.18 126.62,51.18 v126.75,51.05 | J12.4 122.43,44.96 124.84,44.96 | 124.84,44.96 v125.86,44.96 | U7.7 124.84,44.96 | J11.3 97.4,42.04 v97.66,41.78 | v165.1,42.54 165.6,43.04 J10.3 | v139.19,39.37 138.81,38.99 v136.02,38.99
  Bottom 0.254: v108.08,38.99 98.17,38.99 97.66,39.5 v97.66,41.78 | v125.86,44.96 125.86,43.05 126.62,42.29 133.22,42.29 136.02,39.5 v136.02,38.99 132.97,38.99 v110.49,38.99 | v125.86,44.96 | v125.86,44.96 125.86,49.66 126.75,50.55 v126.75,51.05 | v165.1,42.54 165.1,40.26 164.21,39.37 v139.19,39.37
SDA/MOSI2  (via drill 0.35)
  Top 0.254: v27.43,86.49 v25.02,86.49 | J23.2 39.88,98.93 40.13,98.68 43.56,98.68 v43.69,98.55 | J21.4 39.37,92.46 41.78,92.46 | 41.78,92.46 v42.8,92.46 | U11.7 41.78,92.46 | J20.3 14.34,89.54 v14.61,89.28 | v82.04,90.04 82.54,90.54 J19.3 | v56.13,86.87 55.75,86.49 v52.96,86.49
  Bottom 0.254: v25.02,86.49 15.11,86.49 14.61,87 v14.61,89.28 | v42.8,92.46 42.8,90.55 43.56,89.79 50.16,89.79 52.96,87 v52.96,86.49 49.91,86.49 v27.43,86.49 | v42.8,92.46 | v42.8,92.46 42.8,97.16 43.69,98.04 v43.69,98.55 | v82.04,90.04 82.04,87.76 81.15,86.87 v56.13,86.87
SDA/MOSI3  (via drill 0.35)
  Top 0.254: v110.49,86.49 v108.08,86.49 | J32.2 122.94,98.93 123.19,98.68 126.62,98.68 v126.75,98.55 | J30.4 122.43,92.46 124.84,92.46 | 124.84,92.46 v125.86,92.46 | U15.7 124.84,92.46 | J29.3 97.4,89.54 v97.66,89.28 | v165.1,90.04 165.6,90.54 J28.3 | v139.19,86.87 138.81,86.49 v136.02,86.49
  Bottom 0.254: v108.08,86.49 98.17,86.49 97.66,87 v97.66,89.28 | v125.86,92.46 125.86,90.55 126.62,89.79 133.22,89.79 136.02,87 v136.02,86.49 132.97,86.49 v110.49,86.49 | v125.86,92.46 | v125.86,92.46 125.86,97.16 126.75,98.04 v126.75,98.55 | v165.1,90.04 165.1,87.76 164.21,86.87 v139.19,86.87
VIN
  Top 0.508: D11.A 73.77,39.5 J9.PWR
  Bottom 0.508: J9.PWR 67.7,43.2 JP7.1
VIN1
  Top 0.508: D20.A 156.83,39.5 J18.PWR
  Bottom 0.508: J18.PWR 150.76,43.2 JP18.1
VIN2
  Top 0.508: D30.A 73.77,87 J27.PWR
  Bottom 0.508: J27.PWR 67.7,90.69 JP27.1
VIN3
  Top 0.508: D40.A 156.83,87 J36.PWR
  Bottom 0.508: J36.PWR 150.76,90.69 JP36.1

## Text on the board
Bottom: x01 | x01 | x01 | x01
Dimension: Route Out | Route Out | Route Out | Route Out
Milling: v-score | v-score | v-score | v-score | Route Out | Route Out | Route Out | Route Out | Route Out | Route Out | Route Out | Route Out | Route Out | Route Out | Route Out | Route Out | Route Out | Route Out | v-score | Route Out | Route Out | Route Out | Route Out | Route Out | Route Out | Route Out | Route Out | Route Out | Route Out | Route Out | Route Out | Route Out | Route Out | v-score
